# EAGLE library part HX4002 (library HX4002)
Low Noise Regulated Charge Pump in SOT23-6 Source: Datasheet
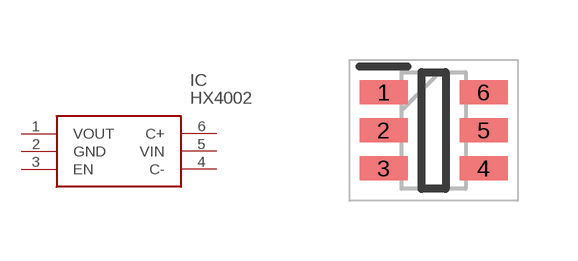
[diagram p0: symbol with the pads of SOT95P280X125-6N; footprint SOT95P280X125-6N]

Designator prefix IC

## HX4002 (Description: Low Noise Regulated Charge Pump in SOT23-6; Height: 1.25mm; Manufacturer_Name: HEXIN; Manufacturer_Part_Number: HX4002)  [SOT95P280X125-6N]
1  VOUT
2  GND
3  EN
4  C-
5  VIN
6  C+

## Footprint SOT95P280X125-6N (pad centres in mm)
SOT-23-6
smd 1.2 x 0.6: 1 -1.25,0.95; 2 -1.25,0; 3 -1.25,-0.95; 4 1.25,-0.95; 5 1.25,0; 6 1.25,0.95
